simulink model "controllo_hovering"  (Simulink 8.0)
settings: Solver=ode45  StartTime=0.0  StopTime=100.0  RelTol=1e-3
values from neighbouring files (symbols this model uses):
  param = [b, d, g, Ix, Iy, Iz, l, m, Jm]    [init.m]
  Rphi = 0.8*tf([0.25 1],[0.0025 1])    [init.m]
  Rpsi = 1.6*tf([0.25 1],[0.0025 1])    [init.m]
  Rtheta = 0.8*tf([0.25 1],[0.0025 1])    [init.m]
  Rx = 10/g*tf([1 1],[0.01 1])    [init.m]
  Ry = -10/g*tf([1 1],[0.01 1])    [init.m]
  Rz = 80*tf([0.25 1],[0.0025 1])    [init.m]
undefined symbols (not defined in the file or in its folder): quadrotor_dynamics, traiettoria_spirale, U2omegaSquare

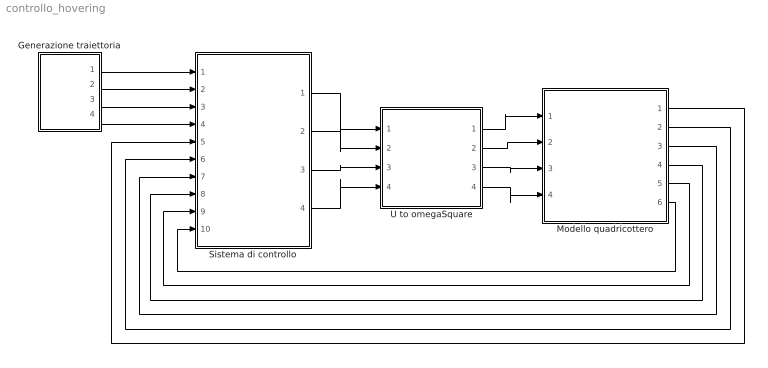
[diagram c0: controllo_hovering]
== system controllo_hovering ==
  Generazione traiettoria : Subsystem
  Modello quadricottero : Subsystem
  Sistema di controllo : Subsystem
  U to omegaSquare : Subsystem
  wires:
  U to omegaSquare/2(omegaSquare2) -> Modello quadricottero/2(omegaSquare2)
  U to omegaSquare/3(omegaSquare3) -> Modello quadricottero/3(omegaSquare3)
  U to omegaSquare/1(omegaSquare1) -> Modello quadricottero/1(omegaSquare1)
  U to omegaSquare/4(omegaSquare4) -> Modello quadricottero/4(omegaSquare4)
  Sistema di controllo/2(U2) -> U to omegaSquare/2(U2)
  Sistema di controllo/1(U1) -> U to omegaSquare/1(U1)
  Sistema di controllo/3(U3) -> U to omegaSquare/3(U3)
  Sistema di controllo/4(U4) -> U to omegaSquare/4(U4)
  Generazione traiettoria/1(xd) -> Sistema di controllo/1(xd)
  Generazione traiettoria/2(yd) -> Sistema di controllo/2(yd)
  Generazione traiettoria/3(zd) -> Sistema di controllo/3(zd)
  Generazione traiettoria/4(psid) -> Sistema di controllo/4(psid)
  Modello quadricottero/6(Psi) -> Sistema di controllo/10(psi)
  Modello quadricottero/5(Theta) -> Sistema di controllo/9(theta)
  Modello quadricottero/4(Phi) -> Sistema di controllo/8(phi)
  Modello quadricottero/3(Z) -> Sistema di controllo/7(z)
  Modello quadricottero/2(Y) -> Sistema di controllo/6(y)
  Modello quadricottero/1("X ") -> Sistema di controllo/5(x)

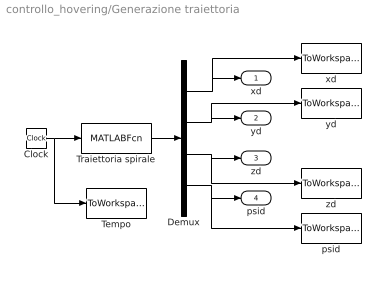
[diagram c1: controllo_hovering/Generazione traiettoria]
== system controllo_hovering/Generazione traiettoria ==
  " psid " : ToWorkspace  VariableName=psid  SampleTime=-1
  " xd " : ToWorkspace  VariableName=xd  SampleTime=-1
  " yd " : ToWorkspace  VariableName=yd  SampleTime=-1
  " zd " : ToWorkspace  VariableName=zd  SampleTime=-1
  Clock : Clock
  Demux : Demux
  Tempo : ToWorkspace  VariableName=t  SampleTime=-1
  Traiettoria spirale : MATLABFcn  MATLABFcn=traiettoria_spirale(u)  OutputDimensions=4
  xd : Outport
  yd : Outport  Port=2
  zd : Outport  Port=3
  psid : Outport  Port=4
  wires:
  Clock/1 -> Tempo/1, Traiettoria spirale/1
  Traiettoria spirale/1 -> Demux/1
  Demux/1 -> " xd "/1, xd/1
  Demux/2 -> " yd "/1, yd/1
  Demux/3 -> " zd "/1, zd/1
  Demux/4 -> " psid "/1, psid/1

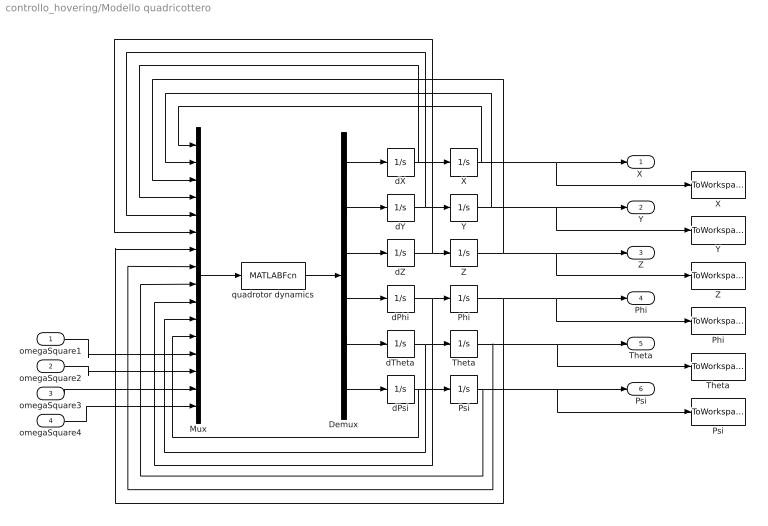
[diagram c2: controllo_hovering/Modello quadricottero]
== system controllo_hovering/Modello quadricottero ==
  omegaSquare1 : Inport
  omegaSquare2 : Inport  Port=2
  omegaSquare3 : Inport  Port=3
  omegaSquare4 : Inport  Port=4
  "  Phi  " : ToWorkspace  VariableName=phi  SampleTime=-1
  "  Psi  " : ToWorkspace  VariableName=psi  SampleTime=-1
  "  Theta  " : ToWorkspace  VariableName=theta  SampleTime=-1
  "  X  " : ToWorkspace  VariableName=x  SampleTime=-1
  "  Y  " : ToWorkspace  VariableName=y  SampleTime=-1
  "  Z  " : ToWorkspace  VariableName=z  SampleTime=-1
  " Phi " : Integrator
  " Psi " : Integrator
  " Theta " : Integrator
  " X " : Integrator
  " Y " : Integrator
  " Z " : Integrator
  Demux : Demux  Outputs=6
  Mux : Mux  Inputs=16
  dPhi : Integrator
  dPsi : Integrator
  dTheta : Integrator
  dX : Integrator
  dY : Integrator
  dZ : Integrator
  quadrotor dynamics : MATLABFcn  MATLABFcn=quadrotor_dynamics(u(1:12),u(13:16),param)  OutputDimensions=6
  "X " : Outport
  Y : Outport  Port=2
  Z : Outport  Port=3
  Phi : Outport  Port=4
  Theta : Outport  Port=5
  Psi : Outport  Port=6
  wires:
  quadrotor dynamics/1 -> Demux/1
  Mux/1 -> quadrotor dynamics/1
  dZ/1 -> Mux/6, " Z "/1
  dPhi/1 -> Mux/10, " Phi "/1
  dTheta/1 -> Mux/11, " Theta "/1
  dPsi/1 -> Mux/12, " Psi "/1
  Demux/1 -> dX/1
  Demux/2 -> dY/1
  Demux/3 -> dZ/1
  Demux/4 -> dPhi/1
  Demux/5 -> dTheta/1
  Demux/6 -> dPsi/1
  " X "/1 -> "X "/1, "  X  "/1, Mux/1
  " Y "/1 -> "  Y  "/1, Y/1, Mux/2
  " Z "/1 -> Z/1, "  Z  "/1, Mux/3
  dX/1 -> Mux/4, " X "/1
  dY/1 -> Mux/5, " Y "/1
  " Phi "/1 -> Phi/1, "  Phi  "/1, Mux/7
  " Theta "/1 -> Theta/1, "  Theta  "/1, Mux/8
  " Psi "/1 -> Psi/1, "  Psi  "/1, Mux/9
  omegaSquare1/1 -> Mux/13
  omegaSquare2/1 -> Mux/14
  omegaSquare3/1 -> Mux/15
  omegaSquare4/1 -> Mux/16

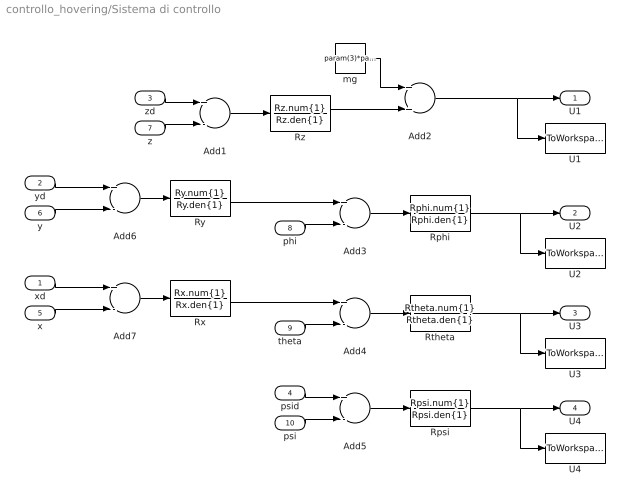
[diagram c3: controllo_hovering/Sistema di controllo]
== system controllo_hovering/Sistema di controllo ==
  xd : Inport
  yd : Inport  Port=2
  zd : Inport  Port=3
  psid : Inport  Port=4
  x : Inport  Port=5
  y : Inport  Port=6
  z : Inport  Port=7
  phi : Inport  Port=8
  theta : Inport  Port=9
  psi : Inport  Port=10
  " U1 " : ToWorkspace  VariableName=U1  SampleTime=-1
  " U2 " : ToWorkspace  VariableName=U2  SampleTime=-1
  " U3 " : ToWorkspace  VariableName=U3  SampleTime=-1
  " U4 " : ToWorkspace  VariableName=U4  SampleTime=-1
  Add{1,3..7} (6 alike) : Sum  Inputs=+-
  Add2 : Sum
  Rphi : TransferFcn  Numerator=Rphi.num{1}  Denominator=Rphi.den{1}
  Rpsi : TransferFcn  Numerator=Rpsi.num{1}  Denominator=Rpsi.den{1}
  Rtheta : TransferFcn  Numerator=Rtheta.num{1}  Denominator=Rtheta.den{1}
  Rx : TransferFcn  Numerator=Rx.num{1}  Denominator=Rx.den{1}
  Ry : TransferFcn  Numerator=Ry.num{1}  Denominator=Ry.den{1}
  Rz : TransferFcn  Numerator=Rz.num{1}  Denominator=Rz.den{1}
  mg : Constant  Value=param(3)*param(8)
  U1 : Outport
  U2 : Outport  Port=2
  U3 : Outport  Port=3
  U4 : Outport  Port=4
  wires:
  Add1/1 -> Rz/1
  mg/1 -> Add2/1
  Rz/1 -> Add2/2
  z/1 -> Add1/2
  zd/1 -> Add1/1
  Add3/1 -> Rphi/1
  phi/1 -> Add3/2
  Add4/1 -> Rtheta/1
  theta/1 -> Add4/2
  Add5/1 -> Rpsi/1
  psi/1 -> Add5/2
  psid/1 -> Add5/1
  Add6/1 -> Ry/1
  Add7/1 -> Rx/1
  xd/1 -> Add7/1
  x/1 -> Add7/2
  yd/1 -> Add6/1
  y/1 -> Add6/2
  Ry/1 -> Add3/1
  Rx/1 -> Add4/1
  Add2/1 -> " U1 "/1, U1/1
  Rphi/1 -> " U2 "/1, U2/1
  Rtheta/1 -> " U3 "/1, U3/1
  Rpsi/1 -> " U4 "/1, U4/1

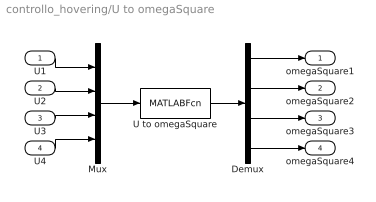
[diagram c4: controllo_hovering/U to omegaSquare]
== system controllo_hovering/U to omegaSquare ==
  U1 : Inport
  U2 : Inport  Port=2
  U3 : Inport  Port=3
  U4 : Inport  Port=4
  Demux : Demux
  Mux : Mux
  U to omegaSquare : MATLABFcn  MATLABFcn=U2omegaSquare(u(1:4),param)  OutputDimensions=4
  omegaSquare1 : Outport
  omegaSquare2 : Outport  Port=2
  omegaSquare3 : Outport  Port=3
  omegaSquare4 : Outport  Port=4
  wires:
  U2/1 -> Mux/2
  U1/1 -> Mux/1
  U3/1 -> Mux/3
  U4/1 -> Mux/4
  Mux/1 -> U to omegaSquare/1
  U to omegaSquare/1 -> Demux/1
  Demux/2 -> omegaSquare2/1
  Demux/3 -> omegaSquare3/1
  Demux/4 -> omegaSquare4/1
  Demux/1 -> omegaSquare1/1
